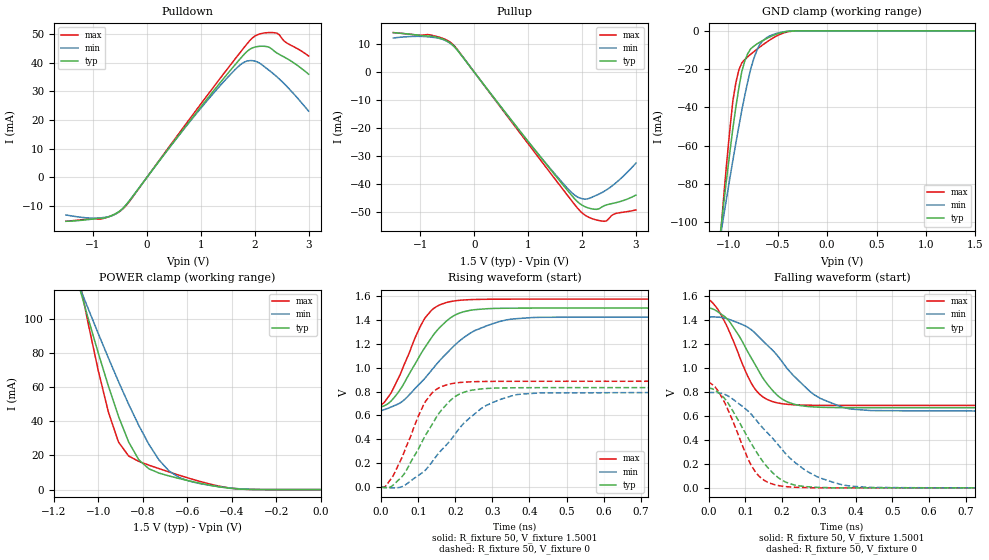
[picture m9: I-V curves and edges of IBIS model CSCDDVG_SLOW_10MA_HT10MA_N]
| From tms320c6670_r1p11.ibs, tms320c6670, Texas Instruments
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|   Model Cell CSCDDVG_SLOW_10MA_HT10MA_N
|SLOW_10MA
[Model]   CSCDDVG_SLOW_10MA_HT10MA_N
Model_type   I/O
Polarity   Non-Inverting
Enable   Active-Low
Cref =  4.0000pF
Rref =  100.0000M
Vref =  0V
Vmeas =  0.75
C_comp   1.5249p   1.4275p   1.6205p
|[mode_tieoffpin] SR0=0  SR1=1 I0=0 I1=1 I2=1
[Model Spec]
Vinl   0.6125   0.6125   0.6125
Vinh   0.9625   0.9625   0.9625
D_overshoot_high 1.95 1.95 1.95
D_overshoot_low -0.3 -0.3 -0.3
D_overshoot_time 1E-9 1E-9 1E-9
S_overshoot_high 1.575 1.575 1.575
S_overshoot_low 0 0 0
[Receiver Thresholds]
Vcross_low = 0.5625V
Vcross_high = 0.9375V
Vdiff_ac = +350mV
Vdiff_dc = +200mV
Tdiffslew_ac = 350ps
[Add Submodel]|Submodel_name Mode
DIFF_HT_TH_10MA Non-Driving
[Temperature Range]   25   105   -40
[Voltage Range]   1.5   1.425   1.575
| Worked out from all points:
|   slope of the pulldown table from 0 to 0.225 V, typ, clamps not added: 39.9 ohm
|   slope of the pullup table from 0 to 0.225 V, typ, clamps not added: 39.8 ohm
|   GND clamp passes 1 mA (typ) near -0.47 V on its own axis
|   POWER clamp passes 1 mA (typ) near -0.42 V on its own axis
|   rising waveform, R_fixture 50, V_fixture 1.5001: 20-80 % time 102ps typ, 147ps min, 75.6ps max; typ from 0.669 V to 1.5 V
|   rising waveform, R_fixture 50, V_fixture 0: 20-80 % time 96.4ps typ, 137ps min, 73ps max; typ from 0 V to 0.834 V
|   falling waveform, R_fixture 50, V_fixture 1.5001: 20-80 % time 99.2ps typ, 145ps min, 75.9ps max; typ from 1.5 V to 0.669 V
|   falling waveform, R_fixture 50, V_fixture 0: 20-80 % time 101ps typ, 148ps min, 73.9ps max; typ from 0.833 V to 0 V
[POWER_clamp]
|   voltage   I(typ)   I(min)   I(max)
-1.5V     321.7mA    260.6mA    415.9mA
-1.076V   114.2mA    115.8mA    116.9mA
-1.061V   107.2mA    110.9mA    107.1mA
-954.6mV  60.59mA    77.06mA    45.35mA
-909.2mV  42.85mA    63.21mA    27.81mA
-863.7mV  27.9mA     49.99mA    19.69mA
-818.2mV  17.49mA    37.63mA    16.52mA
-772.8mV  12.19mA    26.53mA    14.33mA
-681.9mV  7.985mA    10.89mA    10.33mA
-590.9mV  5.094mA    4.955mA    6.6mA
-363.7mV  298.5uA    465.2uA    297.6uA
0V        1.518nA    24.08nA    367.8pA
[Pulldown]
|   voltage   I(typ)   I(min)   I(max)
-1.5V     -15.29mA   -13.07mA   -15.28mA
-772.8mV  -14.07mA   -13.9mA    -14.11mA
-590.9mV  -12.74mA   -12.86mA   -12.82mA
-409.1mV  -10.08mA   -10.11mA   -10.32mA
1.046V    25.68mA    25.17mA    26.75mA
1.591V    38.31mA    36.75mA    40.25mA
1.818V    43.24mA    40.36mA    45.69mA
1.955V    45.18mA    40.77mA    48.64mA
2.091V    45.77mA    39.91mA    50.06mA
2.273V    45.4mA     37.32mA    50.56mA
2.364V    44.07mA    35.93mA    50.51mA
3V        36.04mA    23.14mA    42.4mA
[Pullup]
|   voltage   I(typ)   I(min)   I(max)
-1.5V     14.1mA     12.18mA    14.13mA
-818.2mV  12.87mA    12.54mA    13.29mA
-590.9mV  11.83mA    11.72mA    12.11mA
-409.1mV  9.844mA    9.773mA    10.15mA
1.227V    -30.36mA   -30.27mA   -31.43mA
1.727V    -42.29mA   -41.55mA   -44.05mA
1.909V    -46.29mA   -44.65mA   -48.54mA
2.046V    -48.11mA   -45.48mA   -51.1mA
2.227V    -49.12mA   -44.44mA   -52.74mA
2.409V    -47.87mA   -42.71mA   -53.43mA
2.591V    -46.92mA   -40.26mA   -50.87mA
3V        -44.02mA   -32.61mA   -49.35mA
[GND_clamp]
|   voltage   I(typ)   I(min)   I(max)
-1.5V     -310.1mA   -250.5mA   -402.5mA
-1.076V   -103.6mA   -106.2mA   -105.2mA
-1.046V   -89.81mA   -96.36mA   -86.02mA
-954.6mV  -51.22mA   -67.87mA   -36.88mA
-924.3mV  -40.08mA   -58.86mA   -27.29mA
-863.7mV  -21.24mA   -41.56mA   -16.73mA
-833.4mV  -15.8mA    -33.75mA   -15.03mA
-772.8mV  -9.345mA   -19.75mA   -12.19mA
-712.2mV  -6.928mA   -10.35mA   -9.704mA
-621.3mV  -4.261mA   -3.896mA   -6.225mA
-409.1mV  -337.1uA   -289.1uA   -618.9uA
1.5V      1.518nA    257.2nA    299pA
[Ramp]
| variable   typ   min   max
dV/dt_f   0.665312/0.14716328n   0.63012/0.22330251n   0.71/0.11480851n
dV/dt_r 0.67173512/0.14256136n 0.64143768/0.21543312n 0.71245768/0.10990193n
R_load = 50
[Rising Waveform]
R_fixture = 50
V_fixture = 1.5001
V_fixture_min = 1.425
V_fixture_max = 1.575
|   time   V(typ)   V(min)   V(max)
0s        669.3mV    639.1mV    688.4mV
26.95ps   722.1mV    671.4mV    790.8mV
44.61ps   788.4mV    694.7mV    901.6mV
93.68ps   1.044V     833.9mV    1.267V
119.5ps   1.177V     917.6mV    1.423V
144.3ps   1.289V     1.011V     1.502V
175.2ps   1.389V     1.116V     1.546V
250.5ps   1.486V     1.309V     1.572V
349.2ps   1.499V     1.407V     1.575V
1.091ns   1.5V       1.425V     1.575V
[Rising Waveform]
R_fixture = 50
V_fixture = 0
V_fixture_min = 0
V_fixture_max = 0
|   time   V(typ)   V(min)   V(max)
0s        0V         0V         0V
29.33ps   9.547mV    -6.305mV   80.41mV
58.47ps   96.39mV    7.323mV    266mV
120.1ps   437.3mV    144.2mV    720.9mV
145.7ps   569mV      246.4mV    811.2mV
181.4ps   709.7mV    372.4mV    860.5mV
217.6ps   788.4mV    516.8mV    877.8mV
270.2ps   822.7mV    659.1mV    884.7mV
368.9ps   832.6mV    776.2mV    886.6mV
1.099ns   833.5mV    794.6mV    886.9mV
[Falling Waveform]
R_fixture = 50
V_fixture = 1.5001
V_fixture_min = 1.425
V_fixture_max = 1.575
|   time   V(typ)   V(min)   V(max)
0s        1.499V     1.425V     1.575V
25.52ps   1.468V     1.425V     1.488V
53.89ps   1.398V     1.408V     1.322V
105.7ps   1.141V     1.342V     937.2mV
125.2ps   1.036V     1.296V     830.1mV
180.1ps   792.9mV    1.129V     714.5mV
214.5ps   717.3mV    992.6mV    697mV
285.2ps   675.3mV    781.1mV    688.9mV
381.4ps   669.1mV    660.5mV    687.8mV
1.091ns   668.6mV    638.1mV    687.6mV
[Falling Waveform]
R_fixture = 50
V_fixture = 0
V_fixture_min = 0
V_fixture_max = 0
|   time   V(typ)   V(min)   V(max)
0s        832.6mV    794.3mV    886mV
24.12ps   802.1mV    794mV      817.5mV
48.11ps   728.8mV    774.7mV    684.1mV
108.9ps   408.2mV    637.1mV    231.9mV
127.1ps   315.2mV    574.5mV    134.2mV
180.3ps   109mV      392.4mV    25.85mV
220.6ps   35.36mV    250.8mV    7.842mV
265.9ps   9.9mV      141.2mV    2.068mV
377.7ps   0V         18.16mV    0V
1.099ns   0V         0V         0V
